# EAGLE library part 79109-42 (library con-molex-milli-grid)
RECEPTACAL
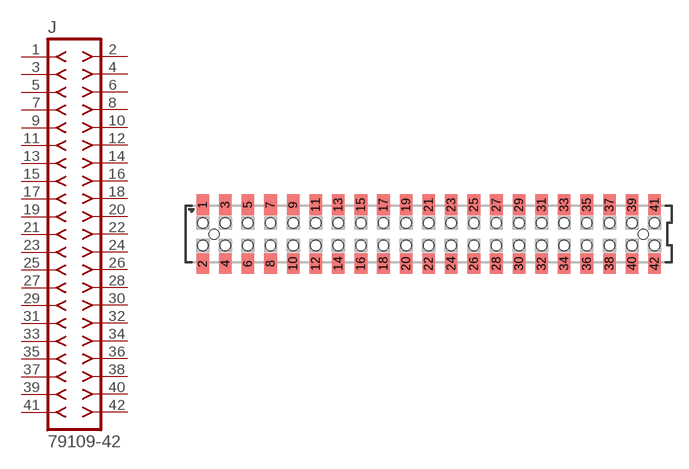
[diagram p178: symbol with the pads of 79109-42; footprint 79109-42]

Designator prefix J

## 79109-42  [79109-42]
1  1  pas
2  2  pas
3  3  pas
4  4  pas
5  5  pas
6  6  pas
7  7  pas
8  8  pas
9  9  pas
10  10  pas
11  11  pas
12  12  pas
13  13  pas
14  14  pas
15  15  pas
16  16  pas
17  17  pas
18  18  pas
19  19  pas
20  20  pas
21  21  pas
22  22  pas
23  23  pas
24  24  pas
25  25  pas
26  26  pas
27  27  pas
28  28  pas
29  29  pas
30  30  pas
31  31  pas
32  32  pas
33  33  pas
34  34  pas
35  35  pas
36  36  pas
37  37  pas
38  38  pas
39  39  pas
40  40  pas
41  41  pas
42  42  pas

## Footprint 79109-42 (pad centres in mm)
RECEPTACAL SMD Dual Row, Vertical, Pass-Thru
smd 1.12 x 1.83: 1 -20,2.6; 2 -20,-2.6; 3 -18,2.6; 4 -18,-2.6; 5 -16,2.6; 6 -16,-2.6; 7 -14,2.6; 8 -14,-2.6; 9 -12,2.6; 10 -12,-2.6; 11 -10,2.6; 12 -10,-2.6; 13 -8,2.6; 14 -8,-2.6; 15 -6,2.6; 16 -6,-2.6; 17 -4,2.6; 18 -4,-2.6; 19 -2,2.6; 20 -2,-2.6; 21 0,2.6; 22 0,-2.6; 23 2,2.6; 24 2,-2.6; 25 4,2.6; 26 4,-2.6; 27 6,2.6; 28 6,-2.6; 29 8,2.6; 30 8,-2.6; 31 10,2.6; 32 10,-2.6; 33 12,2.6; 34 12,-2.6; 35 14,2.6; 36 14,-2.6; 37 16,2.6; 38 16,-2.6; 39 18,2.6; 40 18,-2.6; 41 20,2.6; 42 20,-2.6
hole 0.914 at -19,0
hole 0.914 at -20,1
hole 0.914 at -20,-1
hole 0.914 at -18,-1
hole 0.914 at -18,1
hole 0.914 at -16,-1
hole 0.914 at -16,1
hole 0.914 at 19,0
hole 0.914 at -14,1
hole 0.914 at -14,-1
hole 0.914 at -12,1
hole 0.914 at -12,-1
hole 0.914 at -10,1
hole 0.914 at -10,-1
hole 0.914 at -8,1
hole 0.914 at -8,-1
hole 0.914 at -6,-1
hole 0.914 at -6,1
hole 0.914 at -4,1
hole 0.914 at -4,-1
hole 0.914 at -2,1
hole 0.914 at -2,-1
hole 0.914 at 0,1
hole 0.914 at 0,-1
hole 0.914 at 2,-1
hole 0.914 at 2,1
hole 0.914 at 4,1
hole 0.914 at 6,1
hole 0.914 at 8,1
hole 0.914 at 4,-1
hole 0.914 at 6,-1
hole 0.914 at 8,-1
hole 0.914 at 10,-1
hole 0.914 at 12,-1
hole 0.914 at 14,-1
hole 0.914 at 16,-1
hole 0.914 at 18,-1
hole 0.914 at 10,1
hole 0.914 at 12,1
hole 0.914 at 14,1
hole 0.914 at 16,1
hole 0.914 at 18,1
hole 0.914 at 20,-1
hole 0.914 at 20,1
